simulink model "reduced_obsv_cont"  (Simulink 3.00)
settings: Solver=ode45  StartTime=0.0  StopTime=10.0  RelTol=1e-3
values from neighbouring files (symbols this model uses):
  A = [-0.007  0.012 0 -9.81;-0.128 -0.54 1 0;0.064 0.96 -0.99 0;0 0 1 0]    [Exp7_4.m]    (also in EXP6_10.M = [0 1 0;0 -1.799 6.953;0 0.939 -1.660]; EXP6_8.M = [a11 a12 0 -g;a21 a22 1 0;a31 a31 a33 0;0 1 0 0]; EXP6_9.m = [a11 a12 0 -g;a21 a22 1 0;a31 a31 a33 0;0 1 0 0]; EXP7_1.M = [0 1 0 0;0 0 -mb*g/(1-mb) 0;0 0 0 1;0 0 m2_bar*g/(1-mb) 0])
  B = [0;-0.036;-12.61;0]    [Exp7_4.m]    (also in EXP6_10.M = [0 0;-28.97 -6.453;-0.174 -0.230]; EXP6_8.M = [b1;b2;b3;0]; EXP6_9.m = [b1;b2;b3;0]; EXP7_1.M = [0;1/((m+M)*(1-mb));0;-m2_bar/((m+M)*(1-mb))])
  C = [1 0 0 0;0 1 0 0]    [Exp7_4.m]    (also in EXP6_8.M = [1 0 0 0]; EXP6_9.m = [1 0 0 0]; EXP7_1.M = [1 0 0 0]; EXP7_2.M = [1 0 0 0;0 0 1 0])
  D = [-10 0;0 -10]    [Exp7_4.m]    (also in EXP6_8.M = 0; EXP7_2.M; EXP7_21.m)
  F1 = F(:,1:2)    [Exp7_4.m]    (also in EXP7_2.M; EXP7_21.m)
  F2 = F(:,3:4)    [Exp7_4.m]    (also in EXP7_2.M; EXP7_21.m)
  K = [0.922 -6.5955 -2.35 -8.977]    [Exp7_4.m]    (also in EXP6_10.M = Q*inv(V); EXP6_8.M = acker(A,B,P); EXP6_9.m = acker(A_bar,B_bar,P); EXP7_3.M = acker(A,B,Pc))
  R = L*B    [Exp7_4.m]    (also in EXP7_2.M; EXP7_21.m; GAIN_CAL.M = B*inv(R2)*B')
  T = A12_taw+L_taw*A22_taw-D*L_taw    [Exp7_4.m]    (also in EXP7_2.M; EXP7_21.m)
libraries: simulink3 x12

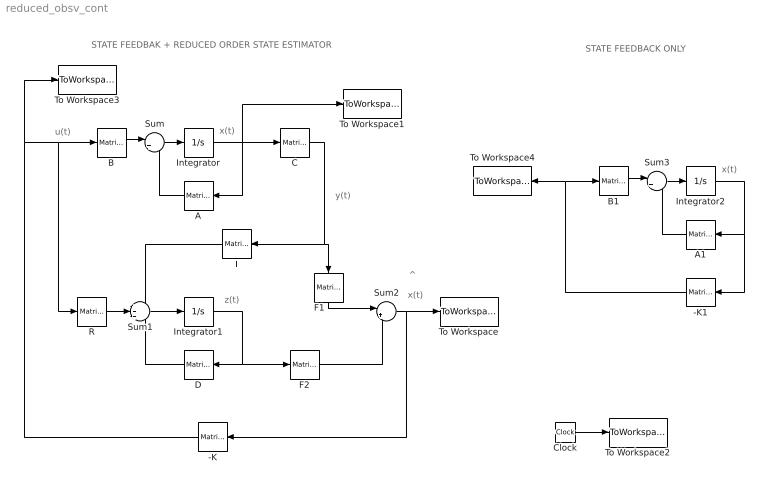
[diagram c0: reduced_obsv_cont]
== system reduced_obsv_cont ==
  note: u(t)
  note: x(t)
  note: y(t)
  note: z(t)
  note: x(t)
  note: ^
  note: x(t)
  note: STATE FEEDBACK ONLY
  note: STATE FEEDBAK + REDUCED ORDER STATE ESTIMATOR
  -K : simulink3/Math/Matrix Gain  Orientation=left  K=-K
  -K1 : simulink3/Math/Matrix Gain  Orientation=left  K=-K
  A : simulink3/Math/Matrix Gain  Orientation=left  K=A
  A1 : simulink3/Math/Matrix Gain  Orientation=left  K=A
  B : simulink3/Math/Matrix Gain  K=B
  B1 : simulink3/Math/Matrix Gain  K=B
  C : simulink3/Math/Matrix Gain  K=C
  Clock : Clock
  D : simulink3/Math/Matrix Gain  Orientation=left  K=D
  F1 : simulink3/Math/Matrix Gain  Orientation=down  K=F1
  F2 : simulink3/Math/Matrix Gain  K=F2
  Integrator : Integrator  ExternalReset=none  InitialConditionSource=internal  InitialCondition=[0.15 .2 0 0.1]  LimitOutput=off  UpperSaturationLimit=inf  LowerSaturationLimit=-inf  ShowSaturationPort=off  ShowStatePort=off  AbsoluteTolerance=auto
  Integrator1 : Integrator  ExternalReset=none  InitialConditionSource=internal  InitialCondition=0  LimitOutput=off  UpperSaturationLimit=inf  LowerSaturationLimit=-inf  ShowSaturationPort=off  ShowStatePort=off  AbsoluteTolerance=auto
  Integrator2 : Integrator  ExternalReset=none  InitialConditionSource=internal  InitialCondition=[0.15 .2 0 0.1]  LimitOutput=off  UpperSaturationLimit=inf  LowerSaturationLimit=-inf  ShowSaturationPort=off  ShowStatePort=off  AbsoluteTolerance=auto
  R : simulink3/Math/Matrix Gain  K=R
  Sum : Sum  Inputs=|++  SaturateOnIntegerOverflow=on
  Sum1 : Sum  Inputs=+++  SaturateOnIntegerOverflow=on
  Sum2 : Sum  Inputs=|++  SaturateOnIntegerOverflow=on
  Sum3 : Sum  Inputs=|++  SaturateOnIntegerOverflow=on
  T : simulink3/Math/Matrix Gain  Orientation=left  K=T
  To Workspace : ToWorkspace  VariableName=estim_state  SampleTime=-1  SaveFormat=Matrix
  To Workspace1 : ToWorkspace  VariableName=real_state  SampleTime=-1  SaveFormat=Matrix
  To Workspace2 : ToWorkspace  VariableName=time  SampleTime=-1  SaveFormat=Matrix
  To Workspace3 : ToWorkspace  VariableName=estim_cont  SampleTime=-1  SaveFormat=Matrix
  To Workspace4 : ToWorkspace  VariableName=real_cont  SampleTime=-1  SaveFormat=Matrix
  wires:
  B/1 -> Sum/1
  Sum/1 -> Integrator/1
  Integrator/1 -> C/1, A/1, To Workspace1/1
  Sum1/1 -> Integrator1/1
  R/1 -> Sum1/2
  A/1 -> Sum/2
  D/1 -> Sum1/3
  T/1 -> Sum1/1
  Integrator1/1 -> D/1, F2/1
  F1/1 -> Sum2/1
  F2/1 -> Sum2/2
  C/1 -> F1/1, T/1
  -K/1 -> B/1, R/1, To Workspace3/1
  Sum2/1 -> To Workspace/1, -K/1
  B1/1 -> Sum3/1
  Sum3/1 -> Integrator2/1
  A1/1 -> Sum3/2
  Integrator2/1 -> A1/1, -K1/1
  -K1/1 -> B1/1, To Workspace4/1
  Clock/1 -> To Workspace2/1
